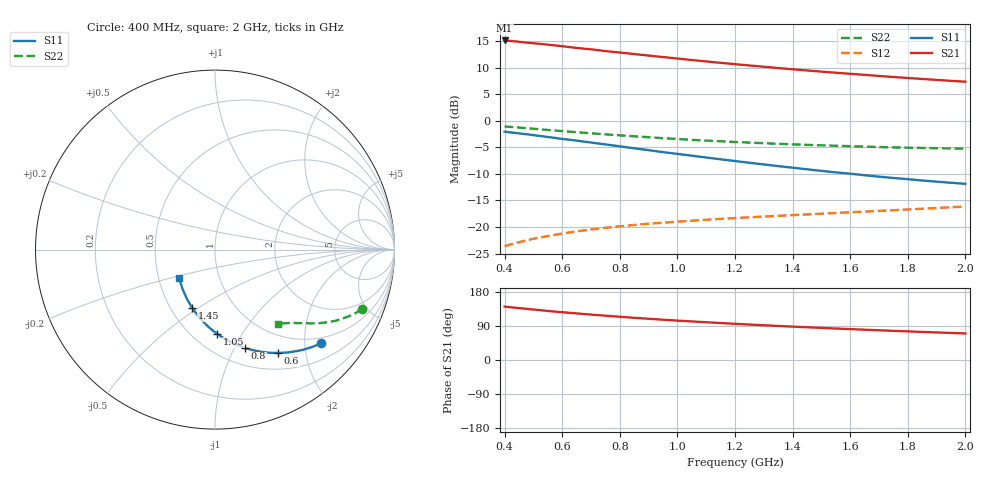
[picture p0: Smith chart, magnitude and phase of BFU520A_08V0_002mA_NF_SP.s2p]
! Filename:  P:\Prog\Test\Noise\ATS_data\Testdata_Net\06 Compressed Noise after Statistics\BFU520A_APG2013_30_A05_08p0V_002mA_NF_CM01_D.sf
! Date/Time: Wed 24/Apr/2013 20:06:19
! BFU520A_APG2013_30_A05_08p0V_1to20mA_NF_CM01_Bias2_R.sf
! Noise Parameter Data File
! BFU520A_APG2013_30_A05_08p0V_1to20mA_NF_CM01
! Date/time: Thu Apr 11 09:33:54 2013
! VAR V_out= 8.000000
! VAR I_out= 2.000000
! VAR V_in= 0.807100
! VAR I_in= 0.021000
! Device data file deembeded for feedlines and parallel
! Original file: \06 Compressed Noise after Statistics\BFU520A_APG2013_30_A05_08p0V_002mA_NF_CM01_R.sf
! Feed-files: PR017V01_150413_Feed1.s2p, PR017V01_150413_Feed2.s2p
! Parallel-file: PR017V01_150413_Par.s2p
# MHz S MA R 50
!  Freq-MHz  S11-mag  S11-arg  S21-mag  S21-arg  S12-mag  S12-arg  S22-mag  S22-arg
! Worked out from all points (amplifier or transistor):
!   37 points, 400 MHz to 2 GHz, reference 50 ohm
!   highest |S21| = 15.1 dB at 400 MHz (marker M1)
!   |S21| within 3 dB of that: start of sweep to 928.5 MHz
!   unconditionally stable (mu >= 1): nowhere
!   at 500 MHz: K = 0.35, MSG = 18.4 dB, |S12| = -22.2 dB
!   at 1.1 GHz: K = 0.69, MSG = 14.9 dB, |S12| = -18.6 dB
!   at 2 GHz: K = 0.98, MSG = 11.7 dB, |S12| = -16.1 dB
!   lowest NFmin = 0.48 dB at 420 MHz
!   S11 on the Smith chart (normalised r, x): 400 MHz: 0.86, -2.37; 600 MHz: 0.73, -1.53; 800 MHz: 0.68, -1.11; 1.05 GHz: 0.65, -0.78; 1.45 GHz: 0.64, -0.47; 2 GHz: 0.64, -0.22
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400  0.7882 -41.4  5.685 141.0  0.0661 66.5  0.8828 -22.0
420  0.7769 -43.3  5.63 139.3  0.0686 65.7  0.8744 -22.9
440  0.7661 -45.1  5.561 137.7  0.07096 64.8  0.8662 -23.6
480  0.744 -48.5  5.407 134.7  0.07536 63.3  0.8486 -25.2
500  0.7318 -50.3  5.354 133.2  0.07753 62.6  0.8405 -25.9
550  0.7034 -54.5  5.195 129.5  0.08234 60.9  0.8185 -27.6
600  0.6748 -58.5  5.024 126.1  0.08683 59.4  0.7989 -29.1
650  0.6502 -62.1  4.837 123.0  0.09108 58.1  0.7802 -30.5
700  0.6233 -65.9  4.692 119.8  0.09476 57.0  0.7616 -31.8
750  0.5988 -69.3  4.52 116.9  0.09833 56.0  0.7446 -32.9
800  0.5743 -72.9  4.379 114.1  0.1016 55.1  0.7282 -34.0
850  0.5503 -76.2  4.236 111.3  0.1046 54.4  0.7132 -35.0
950  0.5065 -82.6  3.97 106.3  0.1099 53.2  0.685 -36.9
1050  0.4688 -88.6  3.722 101.8  0.1147 52.6  0.6605 -38.4
1150  0.4337 -94.5  3.502 97.5  0.1194 52.0  0.6409 -39.8
1200  0.4178 -97.3  3.403 95.5  0.1214 52.0  0.6308 -40.5
1300  0.3881 -102.8  3.217 91.7  0.1255 51.9  0.6147 -41.8
1450  0.3491 -111.2  2.97 86.4  0.1315 52.2  0.5927 -43.6
1500  0.3375 -113.9  2.895 84.7  0.1335 52.4  0.5868 -44.1
1650  0.3071 -122.0  2.698 80.0  0.1398 53.1  0.5714 -45.9
1750  0.2894 -127.7  2.576 76.9  0.144 53.8  0.5614 -46.9
2000  0.2552 -141.4  2.326 70.0  0.156 55.5  0.5453 -49.9
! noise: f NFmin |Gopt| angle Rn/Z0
400  0.5482  0.5114  16.19  0.2182
460  0.5345  0.4943  20.73  0.2129
600  0.631  0.488  25.88  0.2197
800  0.6043  0.469  35.75  0.1801
1000  0.6567  0.4435  48.27  0.1673
1200  0.7013  0.4301  57.37  0.1655
1400  0.7522  0.4018  68.51  0.1467
1600  0.7879  0.3532  80.69  0.1204
1800  0.7121  0.3199  95.17  0.1121
2000  0.7829  0.2489  110.4  0.1061
